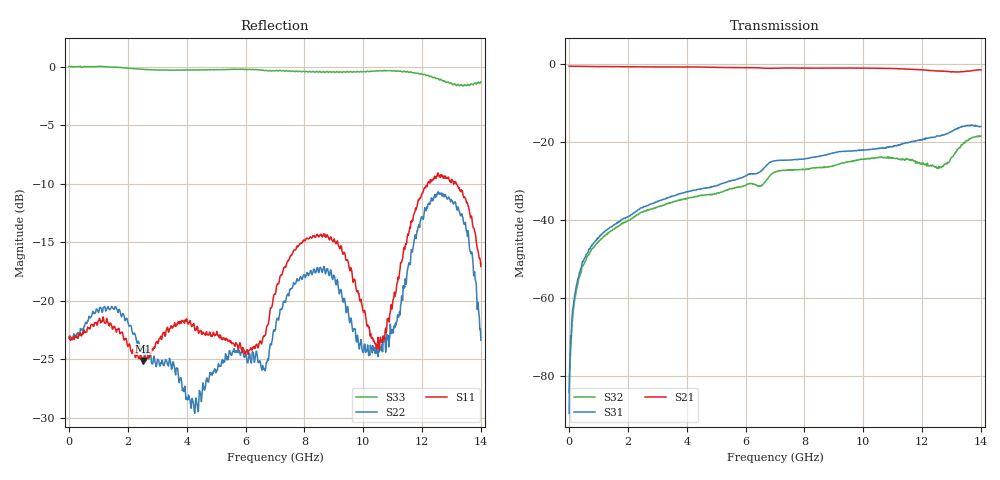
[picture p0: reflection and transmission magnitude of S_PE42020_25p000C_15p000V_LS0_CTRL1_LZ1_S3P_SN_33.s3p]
! Device ID: PE42020
! File Path: z:\PE42020\sparam_retest1\25p000C\3p000\LS_CTRL1_LZ1\PE42020_25p000C_3p000V_3p000V_0p000V_LS_CTRL1_LZ1_S3P_SN_33__2_3.s3p
! Serial: 33
! Lot:
! Temp: 25.000C
! VDD: 15.000
! VSS: -15.000
! Control_Hi: 3.000
! Control_Lo: 0.000
! Logic State: LS_CTRL1_LZ1
! Port 1: RFC
! Port 3: RF2
! Port 4:
! ThroughPath:1-3
! IDD: -0.0020365797
! ISS: 0
! Comment:
#  Hz  S  RI  R  50
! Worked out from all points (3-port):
!   801 points, 300 kHz to 14 GHz, reference 50 ohm
!   strongest paths, dB at 300 kHz, 3.5 GHz, 7 GHz, 10.5 GHz, 14 GHz:
!     S21: -0.6, -0.8, -1.1, -1.1, -1.5
!     S31: -89.6, -33.9, -24.9, -21.7, -16.0
!     S32: -84.2, -35.5, -27.7, -24.1, -18.5
!   lowest |S11| = -25.2 dB at 2.503 GHz (marker M1), VSWR 1.12, Z = 54.6 - j3.52 ohm
!   |S11| at or under -10 dB: start of sweep to 12.19 GHz; 13.0696 GHz to 13.07742 GHz (7.826 MHz wide, 0.0599 % of centre); 13.16 GHz to end of sweep
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300000  0.0703 0.003  0.9342 0.00327  0.000223 0.000445
        0.9335 0.00329  0.0692 0.00343  -8.31e-05 -0.000227
        -3.01e-05 -1.42e-05  4.17e-05 4.55e-05  1.002 0.00335
1.753e8  0.0673 -0.0121  0.9278 -0.0429  -0.00011 0.00099
         0.9293 -0.042  0.0686 -0.0111  -5.52e-05 0.000875
         -2.58e-05 0.00097  -5.62e-05 0.00085  0.9972 -0.0598
5.078e8  0.0675 -0.0328  0.9179 -0.1177  0.000206 0.0031
         0.9191 -0.1175  0.0699 -0.0339  0.000369 0.00281
         0.000282 0.00309  0.000336 0.0027  0.988 -0.1646
2.5028e9  0.045 -0.0321  0.7474 -0.5263  0.00624 0.0131
          0.7471 -0.5282  0.0524 -0.0362  0.00823 0.00971
          0.00623 0.0129  0.00806 0.00964  0.7826 -0.5814
4.3228e9  0.0483 -0.0575  0.4442 -0.7957  0.0172 0.0171
          0.4442 -0.7963  0.0222 -0.0306  0.0189 0.00726
          0.0172 0.017  0.0187 0.00696  0.4125 -0.8776
7.0003e9  0.0672 -0.0829  -0.1145 -0.8727  0.0527 0.0221
          -0.1156 -0.873  0.0661 -0.0357  0.0407 -0.00354
          0.0528 0.0218  0.0409 -0.00334  -0.1591 -0.9462
8.7153e9  0.1035 -0.1559  -0.4626 -0.7488  0.0676 -0.00692
          -0.4642 -0.7486  0.1086 -0.0718  0.0352 -0.0325
          0.0674 -0.00686  0.0352 -0.0319  -0.5448 -0.7763
1.04828e10  0.00265 -0.0647  -0.7456 -0.4683  0.0697 -0.0437
            -0.7445 -0.4661  -0.0348 -0.0547  0.0135 -0.0616
            0.069 -0.0437  0.013 -0.0612  -0.8584 -0.4331
1.26003e10  -0.062 -0.3343  -0.8103 -0.0212  0.0626 -0.1015
            -0.8096 -0.0168  0.0731 -0.2754  -0.00473 -0.0472
            0.0615 -0.1017  -0.00436 -0.0462  -0.8715 -0.1407
1.40003e10  0.0604 -0.1265  -0.8129 0.202  -0.0182 -0.1534
            -0.812 0.2079  0.0541 -0.0408  -0.0581 -0.1004
            -0.0149 -0.157  -0.0586 -0.1033  -0.7435 0.4374
